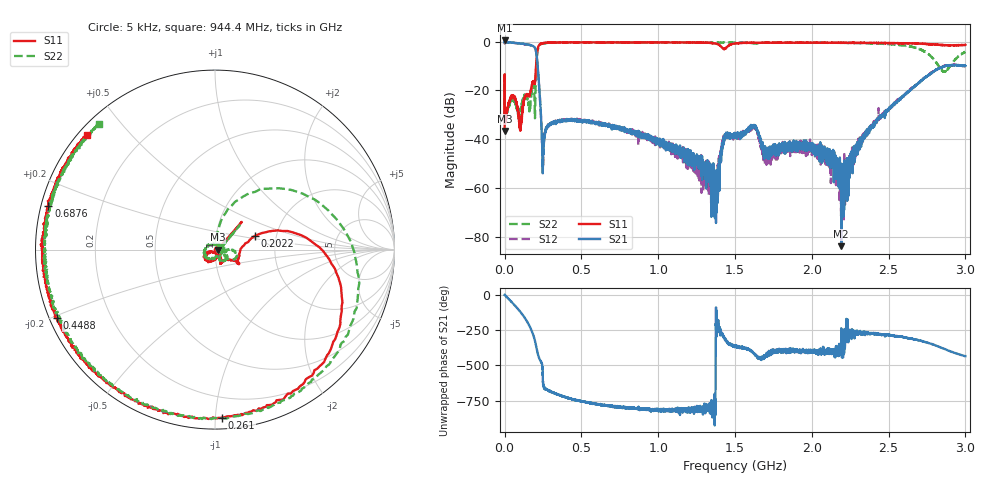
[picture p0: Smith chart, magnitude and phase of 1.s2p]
#  HZ  S  DB  R  50.00
! Rohde & Schwarz Vector Network Analyzer
! Rohde-Schwarz,ZNL6-2Port,1323001206101378,1.50.1.34-21.10.1.104
! Created: UTC 6/16/2023, 6:29:46 AM
! freq[Hz]  db:S11  ang:S11  db:S21  ang:S21  db:S12  ang:S12  db:S22  ang:S22
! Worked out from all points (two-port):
!   5001 points, 5 kHz to 3 GHz, reference 50 ohm
!   highest |S21| = 0.43 dB at 605 kHz (marker M1); lowest = -83.6 dB at 2.192 GHz (marker M2)
!   |S21| within 3 dB of the highest: start of sweep to 197.6 MHz
!   lowest |S11| = -36.5 dB at 5 kHz (marker M3), VSWR 1.03, Z = 51.5 + j0.0408 ohm
!   |S11| at or under -10 dB: start of sweep to 204.6 MHz
!   |S22| runs from -33.4 to -0.3 dB; largest |S21 - S12| = 0.14
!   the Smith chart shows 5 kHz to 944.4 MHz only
!   S11 on the Smith chart (normalised r, x): 5 kHz: 1.03, +0.00; 202.2 MHz: 1.55, +0.25; 261 MHz: 0.07, -1.04; 448.8 MHz: 0.02, -0.21; 687.6 MHz: 0.02, +0.13; 944.4 MHz: 0.02, +0.38
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5000  -36.54 1.5  -0.19 -0.1  -0.20 0.1  -30.89 4.3
604999  -13.37 46.0  0.43 1.9  -0.83 0.5  -14.29 44.6
7.500488e7  -24.39 -148.0  -0.62 -85.8  -0.66 -86.5  -26.35 168.5
1.032048e8  -36.31 -90.8  -0.82 -121.8  -0.81 -122.9  -27.56 44.9
1.356048e8  -22.29 -66.4  -1.08 -170.8  -1.14 -171.4  -21.72 -46.8
1.764047e8  -18.25 -28.2  -1.62 105.1  -1.67 104.7  -20.47 -0.3
2.022047e8  -12.54 19.0  -3.33 12.3  -3.38 11.2  -17.18 79.5
2.286046e8  -1.17 -47.2  -21.69 -97.5  -21.71 -99.3  -1.44 -21.0
2.610046e8  -0.57 -87.6  -37.99 56.0  -37.14 57.3  -0.65 -70.2
4.488043e8  -0.34 -156.6  -32.15 -21.8  -32.36 -24.5  -0.47 -153.4
5.004042e8  -0.34 -166.8  -32.49 -32.5  -32.37 -38.5  -0.43 -164.8
6.876039e8  -0.36 165.4  -34.32 -67.2  -34.29 -71.3  -0.47 164.4
9.444034e8  -0.38 138.3  -39.58 -86.6  -38.03 -96.7  -0.42 132.8
1.000203e9  -0.34 133.0  -40.45 -94.0  -40.86 -97.2  -0.43 126.8
1.375203e9  -0.85 93.9  -63.48 155.6  -68.23 -168.3  -0.41 88.7
1.430403e9  -3.05 96.3  -39.95 56.2  -39.46 67.2  -0.42 83.4
1.500002e9  -0.79 96.2  -38.50 -4.1  -38.74 1.8  -0.39 76.4
2.000402e9  -0.48 49.8  -42.57 -32.1  -43.54 -37.1  -0.43 27.2
2.191801e9  -0.49 33.2  -83.60 122.7  -53.46 3.9  -0.56 5.8
2.500201e9  -0.64 5.1  -28.30 75.8  -27.21 72.9  -1.06 -37.0
2.8074e9  -1.23 -25.4  -11.58 1.3  -11.66 0.1  -8.30 -147.1
3e9  -1.38 -40.6  -9.93 -75.5  -10.05 -75.9  -4.23 10.8
